| IBIS file generated by GenIBIS.pl Version 3.20?
|   centaurus
[IBIS ver]   4.1
[File name]   sprm555a.ibs
[File Rev]   1.0
[Date]   Mon Mar 12, 2012, 13:6:18
[Source]   Data created at Texas Instruments
[Notes]   Checked with IBISCHK5.0.0 with the following exceptions...
   68 warnings. These warnings can be waived.
   Models generated for the following conditions...
   Industrial temperature range -40C to 125C
   Max supply tolerance 10%
   Some pins may contain selectors which are not valid options
   for that particular pin
   Please refer to the device datasheet for information on picking
   the correct selector model, which depends on various software
   register configurations.
   Some pins are modeled as IO or tri-state for output mode
[Disclaimer] Please be aware that in the absence of a written agreement,
   Texas Instruments (TI) assumes no liability for: 1) the
   accuracy of the IBIS models provided to your company, 2) the
   proper functioning of these IBIS models in your design or for
   any resulting applications, or, 3) infringement of patents,
   copyrights, or intellectual property rights resulting from
   your use of these IBIS models. TI provides IBIS models as a
   service to our customers and therefore reserves the right to
   limit distribution of the IBIS models.
[Copyright]   Property of Texas Instruments Incorporated. Unauthorised
   reproduction and/or distribution is strictly prohibited. This
   product is protected under copyright law and trade secret law
   as an unpublished work. Created 2010,(C) Copyright 2010,
   Texas Instruments Incorporated., All Rights Reserved. These
   commodities are under the U.S. Government distribution license
   control.As such,they are not to be re-exported without the
   prior approval of the U.S. Department of Commerce.
|   Component centaurus
[Component]   centaurus
[Manufacturer]   Texas Instruments.
| Source IO level model revisions
|Model   Revision   Date
|BC1833DV40DCPBFBP18LL_SSDHH   1.1   May 27, 2010
|IQ1833DVTCKPBFBP18LL_SSDHH   1.1   May 27, 2010
|BCSHTLTCSCDVPBFZ_SSGFV   1.0   May 31, 2010
|BC1833DV40DCMLBPBFBP18LL_SSDHH   1.1   May 27, 2010
|BCSHTLTCSCDDVPBFZ_SSGFV   1.0   May 31, 2010
|BC1833DV40DCPBFBP18LL_SSDHV   1.1   May 27, 2010
|IHHV1833DVHYP18LL_SSDHH   1.1   May 27, 2010
[Package]
|   typ   min   max
R_pkg   1.068   2.06E-1   1.93E0
L_pkg   3.135E-009   9.00E-10   5.37E-9
C_pkg   2.2305E-012   6.21E-13   3.84E-12
[Pin]   signal_name   model_name   R_pin   L_pin   C_pin
R5   AUD_CLKIN1   Selector_4   9.45E-1   3.06E-9   1.21E-12
H1   AUD_CLKIN2   Selector_4   1.37E0   3.69E-9   1.87E-12
L5   AUD_CLKIN0   Selector_4   6.71E-1   2.16E-9   1.01E-12
R1   AUXOSC_MXI   NC
T1   AUXOSC_MXO   NC
AC22   CAM_D[5]   Selector_4   6.39E-1   1.94E-9   1.07E-12
AB17   CAM_D[7]   Selector_4   1.03E0   3.13E-9   1.41E-12
J7   CLKIN32   Selector_4   3.20E-1   1.40E-9   8.51E-13
AG6   DCAN0_RX   Selector_11  1.16E0   3.22E-9   1.76E-12
AH6   DCAN0_TX   Selector_11  1.31E0   3.47E-9   1.75E-12
B27   DDR[0]_VTP   NC
D2   DDR[1]_DQS[0]N   Selector_5   1.36E0   3.45E-9   1.85E-12
G18   DDR[0]_ODT[0]   Selector_9   1.23E0   3.23E-9   1.73E-12
B19   DDR[0]_A[0]   Selector_9   1.26E0   3.41E-9   1.56E-12
G12   DDR[1]_CS[0]N   Selector_9   1.13E0   3.21E-9   1.57E-12
B10   DDR[1]_A[12]   Selector_9   1.12E0   3.01E-9   1.70E-12
A22   DDR[0]_D[27]   Selector_2   1.26E0   3.33E-9   1.71E-12
B21   DDR[0]_DQS[3]   Selector_5   1.33E0   3.47E-9   1.55E-12
F14   DDR[1]_BA[0]   Selector_9   1.17E0   3.16E-9   1.49E-12
B7   DDR[1]_D[23]   Selector_2   1.30E0   3.46E-9   1.64E-12
A23   DDR[0]_DQS[2]N   Selector_5   1.43E0   3.76E-9   1.79E-12
D21   DDR[0]_D[30]   Selector_2   1.20E0   3.62E-9   1.70E-12
E26   DDR[0]_D[2]   Selector_2   1.53E0   3.78E-9   1.83E-12
F15   DDR[0]_BA[0]   Selector_9   1.25E0   3.63E-9   1.66E-12
F21   DDR[0]_D[25]   Selector_2   1.28E0   3.44E-9   1.85E-12
B17   DDR[0]_A[5]   Selector_9   1.20E0   3.20E-9   1.80E-12
C18   DDR[0]_CASN   Selector_9   1.22E0   3.31E-9   1.69E-12
A11   DDR[1]_A[11]   Selector_9   1.13E0   3.02E-9   1.56E-12
C27   DDR[0]_D[8]   Selector_2   1.55E0   4.01E-9   2.08E-12
C26   DDR[0]_D[10]   Selector_2   1.60E0   4.13E-9   2.02E-12
E28   DDR[0]_DQM[0]   Selector_9   1.55E0   3.87E-9   1.90E-12
D23   DDR[0]_D[20]   Selector_2   1.33E0   3.53E-9   1.94E-12
A3   DDR[1]_DQS[1]N   Selector_5   1.52E0   3.80E-9   1.90E-12
E2   DDR[1]_D[2]   Selector_2   1.34E0   3.62E-9   1.77E-12
C28   DDR[0]_D[7]   Selector_2   1.57E0   3.88E-9   2.07E-12
A8   DDR[1]_DQS[3]N   Selector_5   1.28E0   3.23E-9   1.64E-12
C25   DDR[0]_D[9]   Selector_2   1.57E0   3.94E-9   3.84E-12
F12   DDR[1]_A[10]   Selector_9   1.14E0   3.17E-9   1.62E-12
F5   DDR[1]_D[4]   Selector_2   1.26E0   3.20E-9   1.84E-12
C20   DDR[0]_D[28]   Selector_2   1.26E0   3.32E-9   1.78E-12
A4   DDR[1]_D[14]   Selector_2   1.43E0   3.72E-9   1.94E-12
C6   DDR[1]_D[20]   Selector_2   1.28E0   3.23E-9   1.79E-12
A26   DDR[0]_DQS[1]N   Selector_5   1.63E0   4.15E-9   1.86E-12
D5   DDR[1]_D[9]   Selector_2   1.53E0   3.76E-9   1.90E-12
B2   DDR[1]_DQM[1]   Selector_9   1.53E0   3.96E-9   1.86E-12
B11   DDR[1]_A[0]   Selector_9   1.18E0   3.24E-9   1.50E-12
A5   DDR[1]_D[15]   Selector_2   1.46E0   3.76E-9   1.87E-12
C3   DDR[1]_D[10]   Selector_2   1.55E0   3.97E-9   1.96E-12
D17   DDR[0]_A[11]   Selector_9   1.19E0   3.09E-9   1.68E-12
E18   DDR[0]_A[7]   Selector_9   1.27E0   3.80E-9   1.73E-12
G10   DDR[1]_RST   Selector_9   1.07E0   3.11E-9   1.47E-12
E4   DDR[1]_D[5]   Selector_2   1.36E0   3.56E-9   1.91E-12
F26   DDR[0]_D[1]   Selector_2   1.52E0   3.82E-9   1.92E-12
C24   DDR[0]_DQM[2]   Selector_9   1.40E0   3.60E-9   1.79E-12
A15   DDR[0]_A[6]   Selector_9   1.21E0   3.23E-9   1.79E-12
C5   DDR[1]_D[18]   Selector_2   1.33E0   3.41E-9   1.89E-12
D3   DDR[1]_D[6]   Selector_2   1.32E0   3.47E-9   1.71E-12
B6   DDR[1]_DQS[2]N   Selector_5   1.36E0   3.37E-9   1.68E-12
B13   DDR[1]_CLK   Selector_9   1.20E0   3.79E-9   1.56E-12
E17   DDR[0]_A[12]   Selector_9   1.21E0   3.55E-9   1.65E-12
B16   DDR[0]_CLK   Selector_9   1.27E0   3.88E-9   1.54E-12
G20   DDR[0]_D[26]   Selector_2   1.30E0   3.60E-9   1.82E-12
B3   DDR[1]_DQS[1]   Selector_5   1.51E0   3.78E-9   1.67E-12
F4   DDR[1]_DQM[0]   Selector_9   1.26E0   3.24E-9   1.85E-12
D1   DDR[1]_DQS[0]   Selector_5   1.38E0   3.46E-9   1.70E-12
E12   DDR[1]_WEN   Selector_9   1.17E0   3.19E-9   1.55E-12
G11   DDR[1]_CS[1]N   Selector_9   1.19E0   3.21E-9   1.63E-12
C9   DDR[1]_D[28]   Selector_2   1.18E0   2.93E-9   1.74E-12
E23   DDR[0]_D[21]   Selector_2   1.38E0   3.89E-9   1.95E-12
F9   DDR[1]_D[24]   Selector_2   1.18E0   3.06E-9   1.51E-12
E6   DDR[1]_D[21]   Selector_2   1.31E0   3.50E-9   1.96E-12
B20   DDR[0]_D[31]   Selector_2   1.28E0   3.43E-9   1.66E-12
C15   DDR[0]_A[9]   Selector_9   1.21E0   3.27E-9   1.50E-12
G8   DDR[1]_DQM[2]   Selector_9   1.31E0   3.42E-9   1.56E-12
B4   DDR[1]_D[12]   Selector_2   1.42E0   3.61E-9   2.05E-12
C21   DDR[0]_D[29]   Selector_2   1.31E0   3.59E-9   1.80E-12
A24   DDR[0]_D[15]   Selector_2   1.58E0   4.12E-9   1.99E-12
B25   DDR[0]_D[12]   Selector_2   1.52E0   3.83E-9   2.11E-12
D18   DDR[0]_A[2]   Selector_9   1.26E0   3.33E-9   1.74E-12
A9   DDR[1]_A[7]   Selector_9   1.20E0   3.36E-9   1.83E-12
B26   DDR[0]_DQS[1]   Selector_5   1.61E0   4.15E-9   1.82E-12
F3   DDR[1]_D[1]   Selector_2   1.27E0   3.39E-9   1.64E-12
H8   DDR[1]_D[16]   Selector_2   1.27E0   3.24E-9   1.61E-12
B8   DDR[1]_DQS[3]   Selector_5   1.26E0   3.17E-9   1.50E-12
H21   DDR[0]_D[18]   Selector_2   1.36E0   3.61E-9   1.75E-12
B22   DDR[0]_D[23]   Selector_2   1.36E0   3.76E-9   1.86E-12
C17   DDR[0]_WEN   Selector_9   1.25E0   3.38E-9   1.72E-12
E15   DDR[0]_A[3]   Selector_9   1.20E0   3.31E-9   1.53E-12
F16   DDR[0]_A[14]   Selector_9   1.18E0   3.06E-9   1.44E-12
G17   DDR[0]_CS[1]N   Selector_9   1.24E0   3.18E-9   1.66E-12
F25   DDR[0]_D[3]   Selector_2   1.52E0   3.77E-9   1.99E-12
A16   DDR[0]_CLKN   Selector_9   1.24E0   3.58E-9   1.59E-12
H20   DDR[0]_D[24]   Selector_2   1.26E0   3.60E-9   1.64E-12
C8   DDR[1]_D[30]   Selector_2   1.14E0   3.37E-9   1.61E-12
A6   DDR[1]_DQS[2]   Selector_5   1.38E0   3.50E-9   1.70E-12
H10   DDR[1]_ODT[0]   Selector_9   1.07E0   3.17E-9   1.41E-12
G21   DDR[0]_D[19]   Selector_2   1.33E0   3.36E-9   1.67E-12
H19   DDR[0]_ODT[1]   Selector_9   1.13E0   3.36E-9   1.53E-12
B18   DDR[0]_RASN   Selector_9   1.26E0   3.78E-9   1.79E-12
A13   DDR[1]_CLKN   Selector_9   1.17E0   3.42E-9   1.52E-12
F24   DDR[0]_D[4]   Selector_2   1.51E0   3.26E-9   1.93E-12
A25   DDR[0]_D[14]   Selector_2   1.54E0   4.00E-9   2.15E-12
E27   DDR[0]_D[0]   Selector_2   1.52E0   3.88E-9   1.81E-12
A19   DDR[0]_A[10]   Selector_9   1.21E0   3.63E-9   1.98E-12
C23   DDR[0]_D[22]   Selector_2   1.33E0   3.64E-9   1.74E-12
A21   DDR[0]_DQS[3]N   Selector_5   1.36E0   3.50E-9   1.62E-12
A10   DDR[1]_BA[1]   Selector_9   1.18E0   3.24E-9   1.75E-12
F19   DDR[0]_A[1]   Selector_9   1.21E0   3.14E-9   1.73E-12
D15   DDR[0]_A[4]   Selector_9   1.22E0   3.37E-9   1.59E-12
A14   DDR[1]_A[3]   Selector_9   1.14E0   3.29E-9   1.60E-12
C11   DDR[1]_A[2]   Selector_9   1.18E0   3.11E-9   1.71E-12
F20   DDR[0]_DQM[3]   Selector_9   1.28E0   3.28E-9   1.78E-12
A20   DDR[0]_BA[1]   Selector_9   1.25E0   3.57E-9   1.89E-12
F13   DDR[1]_CASN   Selector_9   1.15E0   2.93E-9   1.52E-12
C14   DDR[1]_A[9]   Selector_9   1.12E0   3.10E-9   1.58E-12
E3   DDR[1]_D[0]   Selector_2   1.27E0   3.46E-9   1.69E-12
B5   DDR[1]_D[19]   Selector_2   1.28E0   3.22E-9   2.06E-12
D27   DDR[0]_DQS[0]N   Selector_5   1.50E0   3.79E-9   1.95E-12
B1   DDR[1]_VTP   NC
B28   DDR[0]_DQM[1]   Selector_9   1.59E0   4.20E-9   1.98E-12
C2   DDR[1]_D[8]   Selector_2   1.48E0   3.80E-9   1.95E-12
F18   DDR[0]_CS[0]N   Selector_9   1.21E0   3.27E-9   1.72E-12
B24   DDR[0]_D[16]   Selector_2   1.36E0   3.60E-9   2.00E-12
F8   DDR[1]_D[26]   Selector_2   1.25E0   3.34E-9   1.72E-12
E11   DDR[1]_A[13]   Selector_9   1.16E0   3.23E-9   1.62E-12
B23   DDR[0]_DQS[2]   Selector_5   1.44E0   3.73E-9   1.83E-12
F10   DDR[1]_A[1]   Selector_9   1.15E0   3.10E-9   1.63E-12
A18   DDR[0]_BA[2]   Selector_9   1.19E0   3.57E-9   1.75E-12
A27   DDR[0]_D[11]   Selector_2   1.55E0   3.94E-9   2.00E-12
A7   DDR[1]_D[27]   Selector_2   1.20E0   2.99E-9   1.70E-12
B9   DDR[1]_D[31]   Selector_2   1.21E0   3.14E-9   1.64E-12
D11   DDR[1]_A[14]   Selector_9   1.13E0   3.04E-9   1.53E-12
G9   DDR[1]_DQM[3]   Selector_9   1.20E0   3.12E-9   1.48E-12
D6   DDR[1]_D[22]   Selector_2   1.27E0   3.43E-9   1.86E-12
F17   DDR[0]_A[13]   Selector_9   1.23E0   3.22E-9   1.74E-12
C1   DDR[1]_D[7]   Selector_2   1.33E0   3.40E-9   1.87E-12
D14   DDR[1]_A[6]   Selector_9   1.18E0   3.14E-9   1.50E-12
F11   DDR[1]_ODT[1]   Selector_9   1.18E0   3.30E-9   1.54E-12
D28   DDR[0]_DQS[0]   Selector_5   1.51E0   3.84E-9   1.68E-12
C12   DDR[1]_RASN   Selector_9   1.20E0   3.36E-9   1.65E-12
F7   DDR[1]_D[17]   Selector_2   1.33E0   3.38E-9   1.77E-12
H9   DDR[1]_D[25]   Selector_2   1.22E0   3.29E-9   1.77E-12
F22   DDR[0]_D[17]   Selector_2   1.39E0   3.53E-9   1.87E-12
B12   DDR[1]_A[5]   Selector_9   1.13E0   3.03E-9   1.59E-12
H11   DDR[1]_CKE   Selector_9   1.09E0   3.30E-9   1.54E-12
A2   DDR[1]_D[11]   Selector_2   1.51E0   3.71E-9   2.02E-12
C4   DDR[1]_D[13]   Selector_2   1.49E0   3.88E-9   2.05E-12
B14   DDR[1]_A[4]   Selector_9   1.14E0   3.37E-9   1.65E-12
E1   DDR[1]_D[3]   Selector_2   1.30E0   3.25E-9   1.69E-12
E14   DDR[1]_A[8]   Selector_9   1.17E0   3.23E-9   1.61E-12
G19   DDR[0]_RST   Selector_9   1.13E0   3.36E-9   1.61E-12
H18   DDR[0]_CKE   Selector_9   1.15E0   3.45E-9   1.63E-12
B15   DDR[0]_A[8]   Selector_9   1.26E0   3.50E-9   1.49E-12
D24   DDR[0]_D[13]   Selector_2   1.58E0   4.13E-9   2.13E-12
D12   DDR[1]_BA[2]   Selector_9   1.14E0   3.10E-9   1.76E-12
D26   DDR[0]_D[6]   Selector_2   1.53E0   3.79E-9   1.87E-12
E25   DDR[0]_D[5]   Selector_2   1.56E0   3.85E-9   1.90E-12
D8   DDR[1]_D[29]   Selector_2   1.24E0   3.51E-9   1.57E-12
AH2   DEVOSC_MXI   NC
AH3   DEVOSC_MXO   NC
W6   DEVOSC_WAKE   Selector_4   1.18E0   3.40E-9   1.79E-12
R23   EMAC[0]_MRXD[2]   Selector_4   1.24E0   3.55E-9   1.90E-12
L23   EMAC[0]_MCOL   Selector_4   5.15E-1   1.64E-9   9.49E-13
H22   EMAC[0]_MTXD[2]   Selector_4   1.00E0   2.82E-9   1.33E-12
J22   EMAC[0]_MTXD[6]   Selector_4   8.58E-1   2.59E-9   1.29E-12
J26   EMAC[0]_MRXER   Selector_4   8.69E-1   2.53E-9   1.22E-12
K22   EMAC[0]_MRXDV   Selector_4   7.90E-1   2.39E-9   1.28E-12
J27   EMAC_RMREFCLK   Selector_4   1.08E0   3.17E-9   1.40E-12
H23   EMAC[0]_MTXD[3]   Selector_4   1.02E0   2.91E-9   1.48E-12
T23   EMAC[0]_MRXD[4]   Selector_4   1.33E0   3.72E-9   1.76E-12
F28   EMAC[0]_MRXD[6]   Selector_4   1.30E0   3.58E-9   1.72E-12
J25   EMAC[0]_MRXD[3]   Selector_4   7.51E-1   2.18E-9   1.24E-12
R25   EMAC[0]_MCRS   Selector_4   1.36E0   3.81E-9   1.66E-12
J23   EMAC[0]_MTXEN   Selector_4   5.73E-1   1.75E-9   1.09E-12
F27   EMAC[0]_MTXD[5]   Selector_4   1.14E0   3.17E-9   1.79E-12
H27   EMAC[0]_MRCLK   Selector_4   1.07E0   3.03E-9   1.35E-12
L24   EMAC[0]_MTCLK   Selector_4   6.57E-1   1.98E-9   1.11E-12
G27   EMAC[0]_MRXD[7]   Selector_4   1.10E0   3.05E-9   1.47E-12
H25   EMAC[0]_MTXD[1]   Selector_4   9.03E-1   2.62E-9   1.31E-12
K23   EMAC[0]_GMTCLK   Selector_4   4.74E-1   1.67E-9   9.00E-13
J24   EMAC[0]_MTXD[0]   Selector_4   6.71E-1   2.13E-9   1.04E-12
P23   EMAC[0]_MRXD[1]   Selector_4   9.64E-1   3.09E-9   1.29E-12
G23   EMAC[0]_MTXD[4]   Selector_4   1.05E0   2.99E-9   1.64E-12
H24   EMAC[0]_MTXD[7]   Selector_4   7.06E-1   2.19E-9   1.19E-12
H26   EMAC[0]_MRXD[5]   Selector_4   9.44E-1   2.78E-9   1.47E-12
G28   EMAC[0]_MRXD[0]   Selector_4   1.26E0   3.34E-9   1.63E-12
AG8   EMU0   Selector_11  1.70E0   4.77E-9   1.95E-12
AE11   EMU1   Selector_11  1.27E0   3.77E-9   1.75E-12
AB28   GPMC_D[9]   Selector_4   1.44E0   3.90E-9   1.94E-12
AE28   GPMC_A[18]   Selector_4   1.51E0   4.38E-9   1.95E-12
V23   GPMC_A[17]   Selector_4   6.27E-1   2.03E-9   1.20E-12
AD27   GPMC_A[16]   Selector_4   1.46E0   3.72E-9   1.96E-12
U23   GPMC_D[13]   Selector_4   5.80E-1   1.78E-9   1.06E-12
M26   GPMC_ADVN_ALE   Selector_4   1.19E0   3.50E-9   1.84E-12
AD28   GPMC_A[20]   Selector_4   1.54E0   4.14E-9   2.05E-12
AC28   GPMC_A[21]   Selector_4   1.44E0   4.27E-9   1.92E-12
U26   GPMC_D[0]   Selector_4   8.82E-1   2.85E-9   1.29E-12
Y27   GPMC_D[8]   Selector_4   1.23E0   3.53E-9   1.73E-12
T27   GPMC_OEN_REN   Selector_4   1.00E0   2.82E-9   1.57E-12
AC27   GPMC_A[19]   Selector_4   1.36E0   3.90E-9   1.75E-12
V26   GPMC_D[4]   Selector_4   1.06E0   3.00E-9   1.56E-12
V24   GPMC_D[14]   Selector_4   7.73E-1   2.39E-9   1.21E-12
Y26   GPMC_D[10]   Selector_4   1.02E0   2.85E-9   1.52E-12
U25   GPMC_D[6]   Selector_4   8.49E-1   2.48E-9   1.35E-12
W28   GPMC_WAIT[0]   Selector_4   1.32E0   3.52E-9   1.72E-12
U28   GPMC_WEN   Selector_4   1.22E0   3.45E-9   1.64E-12
AB27   GPMC_A[22]   Selector_4   1.28E0   3.70E-9   1.88E-12
R26   GPMC_CLK   Selector_4   8.74E-1   2.46E-9   1.37E-12
M25   GPMC_CS[2]N   Selector_4   7.19E-1   2.25E-9   1.46E-12
AA28   GPMC_D[5]   Selector_4   1.41E0   3.90E-9   1.97E-12
P25   GPMC_CS[4]N   Selector_4   1.26E0   3.40E-9   1.56E-12
V27   GPMC_D[2]   Selector_4   1.15E0   3.34E-9   1.59E-12
U27   GPMC_BE[0]N_CLE   Selector_4   1.07E0   3.10E-9   1.61E-12
T28   GPMC_CS[0]N   Selector_4   1.82E0   4.91E-9   2.18E-12
U24   GPMC_D[12]   Selector_4   7.10E-1   2.16E-9   1.22E-12
K28   GPMC_CS[1]N   Selector_4   1.34E0   3.33E-9   1.67E-12
V25   GPMC_D[7]   Selector_4   8.64E-1   2.75E-9   1.13E-12
AA26   GPMC_A[23]   Selector_4   1.03E0   3.09E-9   1.59E-12
W27   GPMC_D[3]   Selector_4   1.25E0   3.42E-9   1.67E-12
V28   GPMC_BE[1]N   Selector_4   1.27E0   3.39E-9   1.63E-12
Y25   GPMC_D[15]   Selector_4   9.86E-1   2.75E-9   1.42E-12
Y28   GPMC_D[1]   Selector_4   1.36E0   3.79E-9   1.76E-12
P26   GPMC_CS[3]N   Selector_4   1.32E0   3.69E-9   1.74E-12
AA27   GPMC_D[11]   Selector_4   1.23E0   3.40E-9   1.68E-12
G6   MCA[3]_ACLKX   Selector_4   1.19E0   3.43E-9   1.64E-12
M4   MCA[0]_AXR[6]   Selector_4   6.90E-1   2.20E-9   1.11E-12
N6   MCA[1]_AXR[3]   Selector_4   3.91E-1   1.58E-9   8.55E-13
M6   MCA[0]_AXR[9]   Selector_4   4.26E-1   1.74E-9   1.01E-12
J4   MCA[4]_AXR[1]   Selector_4   9.89E-1   2.89E-9   1.32E-12
H5   MCA[5]_AFSX   Selector_4   1.27E0   3.56E-9   1.84E-12
L1   MCA[0]_AXR[8]   Selector_4   1.09E0   3.11E-9   1.51E-12
H4   MCA[3]_AFSX   Selector_4   8.85E-1   2.60E-9   1.35E-12
L4   MCA[0]_AXR[2]   Selector_4   7.39E-1   2.46E-9   1.21E-12
L3   MCA[0]_AFSX   Selector_4   8.34E-1   2.46E-9   1.33E-12
K1   MCA[0]_AFSR   Selector_4   1.09E0   3.04E-9   1.52E-12
V3   MCA[1]_AFSX   Selector_4   1.69E0   4.83E-9   2.01E-12
J3   MCA[5]_ACLKX   Selector_4   8.04E-1   2.45E-9   1.47E-12
R4   MCA[0]_ACLKX   Selector_4   1.06E0   3.15E-9   1.50E-12
J6   MCA[3]_AXR[3]   Selector_4   6.01E-1   1.98E-9   1.16E-12
U6   MCA[2]_ACLKX   Selector_4   9.32E-1   2.90E-9   1.28E-12
N2   MCA[2]_AXR[0]   Selector_4   8.59E-1   2.52E-9   1.37E-12
H6   MCA[4]_AXR[0]   Selector_4   1.17E0   3.17E-9   1.61E-12
R6   MCA[0]_AXR[4]   Selector_4   8.02E-1   2.45E-9   1.27E-12
K7   MCA[4]_ACLKX   Selector_4   3.11E-1   1.44E-9   8.81E-13
M5   MCA[0]_AXR[3]   Selector_4   5.38E-1   1.93E-9   1.04E-12
H2   MCA[2]_AXR[3]   Selector_4   1.25E0   3.57E-9   1.71E-12
L7   MCA[5]_AXR[0]   Selector_4   3.14E-1   1.39E-9   7.88E-13
J2   MCA[0]_AXR[0]   Selector_4   1.06E0   3.00E-9   1.53E-12
AA5   MCA[2]_AFSX   Selector_4   1.77E0   5.15E-9   2.14E-12
M3   MCA[0]_AXR[5]   Selector_4   6.82E-1   2.23E-9   1.29E-12
R3   MCA[1]_AXR[2]   Selector_4   1.00E0   3.03E-9   1.31E-12
V4   MCA[1]_AXR[0]   Selector_4   1.62E0   4.67E-9   1.93E-12
U5   MCA[1]_ACLKX   Selector_4   1.21E0   3.49E-9   1.49E-12
G1   MCA[3]_AXR[0]   Selector_4   1.16E0   3.34E-9   1.66E-12
J1   MCA[0]_AXR[1]   Selector_4   1.31E0   3.77E-9   1.60E-12
V6   MCA[2]_AXR[1]   Selector_4   1.21E0   3.48E-9   1.52E-12
L6   MCA[5]_AXR[1]   Selector_4   5.44E-1   1.94E-9   1.02E-12
H3   MCA[4]_AFSX   Selector_4   9.61E-1   2.78E-9   1.49E-12
F2   MCA[3]_AXR[2]   Selector_4   1.24E0   3.47E-9   1.81E-12
K2   MCA[0]_ACLKR   Selector_4   1.07E0   3.00E-9   1.51E-12
T6   MCA[1]_AXR[1]   Selector_4   6.28E-1   2.09E-9   1.16E-12
G2   MCA[3]_AXR[1]   Selector_4   1.09E0   3.15E-9   1.62E-12
M1   MCA[1]_ACLKR   Selector_4   1.06E0   3.13E-9   1.40E-12
M2   MCA[1]_AFSR   Selector_4   1.01E0   2.88E-9   1.44E-12
L2   MCA[0]_AXR[7]   Selector_4   1.04E0   2.82E-9   1.44E-12
V5   MCA[2]_AXR[2]   Selector_4   1.30E0   3.96E-9   1.72E-12
H28   MDCLK   Selector_4   1.16E0   3.25E-9   1.72E-12
P24   MDIO   Selector_4   1.06E0   3.29E-9   1.42E-12
H7   NMIN   Selector_1   9.93E-1   2.99E-9   1.47E-12
F1   PORN   Selector_12  1.37E0   3.48E-9   1.78E-12
J5   RESETN   Selector_1   7.19E-1   2.26E-9   1.13E-12
K6   RSTOUTN_WDN_OUTN   Selector_3   5.10E-1   1.65E-9   9.95E-13
AD4   RTCK   Selector_10  1.01E0   2.73E-9   1.35E-12
Y4   SD0_DAT[3]   Selector_4   1.65E0   4.91E-9   2.04E-12
Y6   SD0_CLK   Selector_4   1.41E0   4.09E-9   1.76E-12
N1   SD0_CMD   Selector_4   1.11E0   3.25E-9   1.48E-12
Y3   SD0_DAT[2]_SDRWN   Selector_4   1.77E0   5.01E-9   2.33E-12
R7   SD0_DAT[0]   Selector_4   3.52E-1   1.36E-9   8.89E-13
Y5   SD0_DAT[1]_SDIRQN   Selector_4   1.54E0   4.43E-9   2.06E-12
P3   SD1_CLK   Selector_3   8.83E-1   2.54E-9   1.28E-12
P6   SD1_DAT[3]   Selector_4   5.29E-1   1.77E-9   9.16E-13
P1   SD1_DAT[0]   Selector_4   1.05E0   2.94E-9   1.43E-12
P5   SD1_DAT[1]_SDIRQN   Selector_4   6.41E-1   2.18E-9   9.48E-13
P4   SD1_DAT[2]_SDRWN   Selector_4   7.18E-1   2.35E-9   1.12E-12
P2   SD1_CMD   Selector_4   9.71E-1   2.85E-9   1.75E-12
L25   SD2_DAT[7]   Selector_4   7.41E-1   2.31E-9   1.18E-12
K27   SD2_DAT[2]_SDRWN   Selector_4   1.08E0   3.10E-9   1.51E-12
M23   SD2_SCLK   Selector_4   5.06E-1   1.67E-9   8.92E-13
M24   SD2_DAT[1]_SDIRQN   Selector_4   5.74E-1   1.89E-9   9.89E-13
L26   SD2_DAT[0]   Selector_4   9.09E-1   2.58E-9   1.29E-12
R24   SD2_DAT[4]   Selector_4   1.07E0   3.12E-9   1.52E-12
N23   SD2_DAT[6]   Selector_4   5.87E-1   2.07E-9   1.02E-12
J28   SD2_DAT[3]   Selector_4   1.17E0   3.18E-9   1.57E-12
P22   SD2_DAT[5]   Selector_4   6.18E-1   2.06E-9   1.05E-12
AD6   SPI[0]_SCS[0]N   Selector_11  8.21E-1   2.38E-9   1.33E-12
AF3   SPI[0]_D[1]   Selector_11  1.25E0   3.81E-9   1.77E-12
AD3   SPI[1]_SCS[0]N   Selector_11  1.18E0   3.37E-9   1.69E-12
AA3   SPI[1]_D[1]   Selector_11  1.26E0   3.76E-9   1.76E-12
AC3   SPI[1]_SCLK   Selector_11  1.15E0   3.22E-9   1.60E-12
AC7   SPI[0]_SCLK   Selector_11  7.08E-1   2.19E-9   1.09E-12
AE5   SPI[0]_SCS[1]N   Selector_11  1.02E0   3.18E-9   1.41E-12
AA6   SPI[1]_D[0]   Selector_11  9.30E-1   2.78E-9   1.49E-12
AE3   SPI[0]_D[0]   Selector_11  1.26E0   3.49E-9   1.76E-12
W7   TCLK   Selector_8   5.20E-1   1.72E-9   9.01E-13
T2   TCLKIN   Selector_7   9.60E-1   2.66E-9   1.33E-12
Y7   TDI   Selector_6   8.98E-1   2.78E-9   1.44E-12
AC5   TDO   Selector_3   7.43E-1   2.13E-9   1.08E-12
AA7   TMS   Selector_1   5.16E-1   1.56E-9   9.14E-13
AA4   TRSTN   Selector_1   9.21E-1   2.56E-9   1.27E-12
AF5   UART0_RTSN   Selector_11  1.13E0   3.73E-9   1.53E-12
AH4   UART0_DCDN   Selector_11  1.35E0   3.74E-9   1.80E-12
AE6   UART0_CTSN   Selector_11  1.00E0   2.80E-9   1.47E-12
AG2   UART0_DTRN   Selector_11  1.46E0   3.89E-9   1.96E-12
AG5   UART0_TXD   Selector_10  1.22E0   3.29E-9   1.74E-12
AF4   UART0_RIN   Selector_11  1.24E0   3.23E-9   1.73E-12
AH5   UART0_RXD   Selector_6   1.38E0   3.54E-9   1.79E-12
AG4   UART0_DSRN   Selector_11  1.31E0   3.62E-9   1.80E-12
U4   UART2_RXD   Selector_7   6.85E-1   2.04E-9   1.16E-12
U3   UART2_TXD   Selector_7   9.31E-1   2.65E-9   1.32E-12
AH8   VIN[0]A_D[4]   Selector_11  1.73E0   4.86E-9   2.37E-12
AB20   VIN[0]A_CLK   Selector_11  4.67E-1   1.63E-9   8.90E-13
AH16   VIN[0]A_D[6]   Selector_11  1.13E0   3.05E-9   1.36E-12
AC20   VIN[0]A_HSYNC   Selector_11  5.37E-1   1.76E-9   9.21E-13
AF17   VIN[0]A_D[13]_BD[5]  Selector_11  7.77E-1   2.45E-9   1.33E-12
AA21   VIN[0]A_D[16]   Selector_4   2.06E-1   9.00E-10   6.21E-13
AD20   VIN[0]A_VSYNC   Selector_11  5.69E-1   1.74E-9   1.12E-12
AF9   VIN[0]A_D[0]   Selector_11  1.65E0   4.87E-9   2.00E-12
AB15   VIN[0]A_D[8]_BD[0]   Selector_11  6.48E-1   2.10E-9   1.11E-12
AC21   VIN[0]A_D[22]   Selector_4   5.25E-1   1.69E-9   9.56E-13
AC12   VIN[0]A_D[14]_BD[6]  Selector_11  1.39E0   4.00E-9   1.65E-12
AE18   VIN[0]A_D[21]   Selector_4   1.09E0   3.15E-9   1.48E-12
AE21   VIN[0]A_DE   Selector_11  8.59E-1   2.54E-9   1.28E-12
AF20   VIN[0]A_D[18]   Selector_4   9.07E-1   2.61E-9   1.42E-12
AC14   VIN[0]A_D[15]_BD[7]  Selector_11  9.28E-1   2.74E-9   1.45E-12
AA11   VIN[0]A_D[7]   Selector_11  9.56E-1   2.86E-9   1.37E-12
AG17   VIN[0]A_D[12]_BD[4]  Selector_11  9.68E-1   2.98E-9   1.52E-12
AB11   VIN[0]A_D[1]   Selector_11  1.10E0   3.24E-9   1.59E-12
AG16   VIN[0]A_D[5]   Selector_11  9.22E-1   2.76E-9   1.42E-12
AE12   VIN[0]A_D[3]   Selector_11  1.15E0   3.70E-9   1.73E-12
AB21   VIN[0]A_D[17]   Selector_4   3.27E-1   1.32E-9   7.89E-13
AE17   VIN[0]B_CLK   Selector_11  1.08E0   3.16E-9   1.61E-12
AC17   VIN[0]A_D[20]   Selector_4   9.04E-1   2.79E-9   1.35E-12
AG9   VIN[0]A_D[9]_BD[1]   Selector_11  1.73E0   4.80E-9   2.21E-12
AH17   VIN[0]A_D[11]_BD[3]  Selector_11  1.14E0   3.37E-9   1.56E-12
AA20   VIN[0]A_FLD   Selector_11  3.16E-1   1.20E-9   7.09E-13
AD17   VIN[0]B_FLD   Selector_4   1.33E0   3.66E-9   1.65E-12
AF21   VIN[0]A_D[19]   Selector_4   9.56E-1   2.77E-9   1.46E-12
AC9   VIN[0]A_D[2]   Selector_11  1.43E0   3.96E-9   1.91E-12
AC15   VIN[0]B_DE   Selector_4   1.40E0   3.92E-9   1.75E-12
AC16   VIN[0]A_D[23]   Selector_4   9.46E-1   2.74E-9   1.28E-12
AH9   VIN[0]A_D[10]_BD[2]  Selector_11  1.79E0   5.09E-9   2.32E-12
AE14   VOUT[0]_G_Y_YC[8]   Selector_10  8.04E-1   2.44E-9   1.19E-12
AH7   VOUT[0]_G_Y_YC[2]   Selector_11  1.93E0   5.37E-9   2.28E-12
AE23   VOUT[1]_B_CB_C[1]   Selector_4   1.03E0   2.93E-9   1.31E-12
AF27   VOUT[1]_G_Y_YC[2]   Selector_4   1.61E0   4.28E-9   2.23E-12
AE26   VOUT[1]_G_Y_YC[8]   Selector_4   1.37E0   3.86E-9   1.99E-12
AD14   VOUT[0]_G_Y_YC[7]   Selector_10  6.42E-1   2.10E-9   1.11E-12
Y24   VOUT[1]_R_CR[9]   Selector_4   7.60E-1   2.30E-9   1.18E-12
AC24   VOUT[1]_HSYNC   Selector_4   7.83E-1   2.40E-9   1.33E-12
AF18   VOUT[0]_FLD   Selector_4   1.38E0   3.80E-9   1.71E-12
AE15   VOUT[0]_B_CB_C[3]   Selector_11  7.36E-1   2.26E-9   1.13E-12
AB9   VOUT[0]_R_CR[3]   Selector_11  9.83E-1   3.02E-9   1.36E-12
AC11   VOUT[0]_HSYNC   Selector_10  1.08E0   3.23E-9   1.44E-12
AG26   VOUT[1]_G_Y_YC[5]   Selector_4   1.54E0   4.35E-9   2.07E-12
Y23   VOUT[1]_G_Y_YC[3]   Selector_4   5.65E-1   1.91E-9   1.11E-12
AG28   VOUT[1]_R_CR[3]   Selector_4   1.75E0   4.64E-9   2.18E-12
AB10   VOUT[0]_B_CB_C[7]   Selector_10  1.01E0   3.09E-9   1.41E-12
AE27   VOUT[1]_R_CR[2]   Selector_4   1.53E0   4.13E-9   2.03E-12
AA25   VOUT[1]_R_CR[6]   Selector_4   9.55E-1   2.72E-9   1.42E-12
AA9   VOUT[0]_R_CR[4]   Selector_10  1.02E0   2.74E-9   1.45E-12
AE8   VOUT[0]_R_CR[8]   Selector_10  1.32E0   3.73E-9   1.81E-12
AF26   VOUT[1]_G_Y_YC[7]   Selector_4   1.44E0   3.93E-9   1.83E-12
AA10   VOUT[0]_AVID   Selector_11  9.05E-1   2.70E-9   1.36E-12
AC25   VOUT[1]_B_CB_C[7]   Selector_4   1.02E0   3.18E-9   1.48E-12
AD12   VOUT[0]_CLK   Selector_10  1.08E0   3.11E-9   1.52E-12
AB23   VOUT[1]_FLD   Selector_4   7.19E-1   2.16E-9   1.04E-12
AA8   VOUT[0]_G_Y_YC[6]   Selector_10  9.40E-1   2.96E-9   1.32E-12
AG7   VOUT[0]_B_CB_C[2]   Selector_11  1.67E0   4.70E-9   2.29E-12
W23   VOUT[1]_R_CR[8]   Selector_4   6.12E-1   1.96E-9   1.16E-12
AF25   VOUT[1]_B_CB_C[5]   Selector_4   1.30E0   3.47E-9   1.80E-12
AF14   VOUT[0]_G_Y_YC[9]   Selector_10  8.54E-1   2.59E-9   1.15E-12
AF6   VOUT[0]_R_CR[6]   Selector_10  1.79E0   5.04E-9   2.20E-12
AG25   VOUT[1]_B_CB_C[4]   Selector_4   1.46E0   3.82E-9   1.96E-12
W22   VOUT[1]_G_Y_YC[4]   Selector_4   3.79E-1   1.38E-9   9.41E-13
AF15   VOUT[0]_B_CB_C[8]   Selector_10  8.55E-1   2.61E-9   1.26E-12
AC10   VOUT[0]_B_CB_C[6]   Selector_10  1.11E0   3.24E-9   1.54E-12
AD25   VOUT[1]_B_CB_C[6]   Selector_4   1.11E0   3.16E-9   1.54E-12
AA22   VOUT[1]_R_CR[0]   Selector_4   4.73E-1   1.49E-9   1.04E-12
AH15   VOUT[0]_G_Y_YC[3]   Selector_11  1.09E0   3.13E-9   1.56E-12
AC26   VOUT[1]_R_CR[5]   Selector_4   1.18E0   3.38E-9   1.62E-12
AB8   VOUT[0]_G_Y_YC[4]   Selector_10  1.26E0   3.66E-9   1.77E-12
AC13   VOUT[0]_R_CR[9]   Selector_10  5.66E-1   1.80E-9   1.09E-12
AF8   VOUT[0]_R_CR[5]   Selector_10  1.42E0   3.89E-9   1.85E-12
AB12   VOUT[0]_G_Y_YC[5]   Selector_10  6.75E-1   2.18E-9   1.08E-12
AD11   VOUT[0]_B_CB_C[4]   Selector_10  1.14E0   3.56E-9   1.54E-12
AD23   VOUT[1]_B_CB_C[0]   Selector_4   9.90E-1   2.65E-9   1.29E-12
AG27   VOUT[1]_R_CR[4]   Selector_4   1.65E0   4.42E-9   2.24E-12
AA23   VOUT[1]_VSYNC   Selector_4   6.19E-1   1.92E-9   1.09E-12
AG15   VOUT[0]_B_CB_C[9]   Selector_10  1.03E0   3.17E-9   1.43E-12
AA24   VOUT[1]_B_CB_C[9]   Selector_4   8.07E-1   2.43E-9   1.24E-12
Y22   VOUT[1]_AVID   Selector_4   5.24E-1   1.58E-9   1.02E-12
AF12   VOUT[0]_R_CR[7]   Selector_10  8.96E-1   2.70E-9   1.34E-12
AH25   VOUT[1]_B_CB_C[3]   Selector_4   1.50E0   4.11E-9   1.93E-12
AD9   VOUT[0]_R_CR[2]   Selector_11  1.25E0   3.63E-9   1.68E-12
AH26   VOUT[1]_B_CB_C[8]   Selector_4   1.60E0   4.29E-9   1.91E-12
AC19   VOUT[1]_R_CR[1]   Selector_4   1.08E0   2.98E-9   1.42E-12
AD18   VOUT[1]_G_Y_YC[1]   Selector_4   1.45E0   4.00E-9   1.84E-12
AC18   VOUT[1]_G_Y_YC[0]   Selector_4   1.37E0   3.88E-9   1.74E-12
AD15   VOUT[0]_B_CB_C[5]   Selector_10  6.31E-1   2.13E-9   1.06E-12
AD26   VOUT[1]_G_Y_YC[9]   Selector_4   1.16E0   3.37E-9   1.80E-12
AE24   VOUT[1]_CLK   Selector_4   1.08E0   3.04E-9   1.62E-12
V22   VOUT[1]_R_CR[7]   Selector_4   5.08E-1   1.57E-9   8.43E-13
AH27   VOUT[1]_G_Y_YC[6]   Selector_4   1.74E0   4.63E-9   2.36E-12
AB13   VOUT[0]_VSYNC   Selector_10  7.62E-1   2.37E-9   1.11E-12
AF28   VOUT1_B_CB_C[2]   Selector_4   1.78E0   4.36E-9   2.27E-12
[Diff Pin] inv_pin vdiff   tdelay_typ
D28   D27   200m   NA
B26   A26   200m   NA
B23   A23   200m   NA
B21   A21   200m   NA
D1   D2   200m   NA
B3   A3   200m   NA
A6   B6   200m   NA
B8   A8   200m   NA
|   Usage INPUT#1.8/3.3#X#X#BC1833DV40DCPBFBP18LL_SSDHH.PAD
|   Base model BC1833DV40DCPBFBP18LL_SSDHH
[Model Selector] Selector_1
Model_13 I/O,1.8V,Pull-up/down off,slow,IND,10%
Model_14 I/O,1.8V,Pull-down,fast,IND,10%
Model_15 I/O,1.8V,Pull-down,slow,IND,10%
Model_16 I/O,1.8V,Pull-up,fast,IND,10%
Model_17 I/O,1.8V,Pull-up/down off,fast,IND,10%
Model_18 I/O,1.8V,Pull-up,slow,IND,10%
Model_19 I/O,3.3V,Pull-up/down off,slow,IND,10%
Model_20 I/O,3.3V,Pull-down,fast,IND,10%
Model_21 I/O,3.3V,Pull-down,slow,IND,10%
Model_22 I/O,3.3V,Pull-up,fast,IND,10%
Model_23 I/O,3.3V,Pull-up/down off,fast,IND,10%
Model_24 I/O,3.3V,Pull-up,slow,IND,10%
|   Usage I/O#1.5/1.8#X#X#BCSHTLTCSCDVPBFZ_SSGFV.PAD
|   Base model BCSHTLTCSCDVPBFZ_SSGFV
[Model Selector] Selector_2
Model_100 3-STATE,1.5V,SLOWEST, 7MA,IND,10%
Model_101 3-STATE,1.5V,slow, 10MA,IND,10%
Model_102 3-STATE,1.5V,SLOWEST, 6MA,IND,10%
Model_103 3-STATE,1.5V,slow, 8MA,IND,10%
Model_104 3-STATE,1.5V,slow, 5MA,IND,10%
Model_105 3-STATE,1.5V,SLOWEST, 11MA,IND,10%
Model_106 3-STATE,1.5V,SLOWEST, 10MA,IND,10%
Model_107 3-STATE,1.5V,slow, 9MA,IND,10%
Model_108 3-STATE,1.5V,slow, 12MA,IND,10%
Model_125 3-STATE,1.8V,fast, 12MA,IND,10%
Model_126 3-STATE,1.8V,FASTEST, 5MA,IND,10%
Model_127 3-STATE,1.8V,FASTEST, 9MA,IND,10%
Model_128 3-STATE,1.8V,fast, 5MA,IND,10%
Model_129 3-STATE,1.8V,FASTEST, 7MA,IND,10%
Model_130 3-STATE,1.8V,FASTEST, 6MA,IND,10%
Model_131 3-STATE,1.8V,fast, 9MA,IND,10%
Model_132 3-STATE,1.8V,FASTEST, 11MA,IND,10%
Model_133 3-STATE,1.8V,fast, 7MA,IND,10%
Model_134 3-STATE,1.8V,FASTEST, 10MA,IND,10%
Model_135 3-STATE,1.8V,fast, 6MA,IND,10%
Model_136 3-STATE,1.8V,FASTEST, 8MA,IND,10%
Model_137 3-STATE,1.8V,fast, 11MA,IND,10%
Model_138 3-STATE,1.8V,fast, 10MA,IND,10%
Model_139 3-STATE,1.8V,FASTEST, 12MA,IND,10%
Model_140 3-STATE,1.8V,fast, 8MA,IND,10%
Model_157 3-STATE,1.5V,fast, 12MA,IND,10%
Model_158 3-STATE,1.5V,FASTEST, 5MA,IND,10%
Model_159 3-STATE,1.5V,FASTEST, 9MA,IND,10%
Model_160 3-STATE,1.5V,fast, 5MA,IND,10%
Model_161 3-STATE,1.5V,FASTEST, 7MA,IND,10%
Model_162 3-STATE,1.5V,FASTEST, 6MA,IND,10%
Model_163 3-STATE,1.5V,fast, 9MA,IND,10%
Model_164 3-STATE,1.5V,FASTEST, 11MA,IND,10%
Model_165 3-STATE,1.5V,fast, 7MA,IND,10%
Model_166 3-STATE,1.5V,FASTEST, 10MA,IND,10%
Model_167 3-STATE,1.5V,fast, 6MA,IND,10%
Model_168 3-STATE,1.5V,FASTEST, 8MA,IND,10%
Model_169 3-STATE,1.5V,fast, 11MA,IND,10%
Model_170 3-STATE,1.5V,fast, 10MA,IND,10%
Model_171 3-STATE,1.5V,FASTEST, 12MA,IND,10%
Model_172 3-STATE,1.5V,fast, 9MA,IND,10%
Model_189 INPUT,1.8V,HALFTERM, 12MA,IND,10%
Model_190 INPUT,1.8V,Pull-up/down off,IND,10%
Model_191 INPUT,1.8V,Pull-down,IND,10%
Model_192 INPUT,1.8V,FULLTERM, 5MA,IND,10%
Model_193 INPUT,1.8V,HALFTERM, 5MA,IND,10%
Model_194 INPUT,1.8V,Pull-up,IND,10%
Model_195 INPUT,1.8V,FULLTERM, 9MA,IND,10%
Model_196 INPUT,1.8V,FULLTERM, 7MA,IND,10%
Model_197 INPUT,1.8V,HALFTERM, 9MA,IND,10%
Model_198 INPUT,1.8V,FULLTERM, 6MA,IND,10%
Model_199 INPUT,1.8V,HALFTERM, 7MA,IND,10%
Model_200 INPUT,1.8V,HALFTERM, 6MA,IND,10%
Model_201 INPUT,1.8V,FULLTERM, 11MA,IND,10%
Model_202 INPUT,1.8V,Pull-up/down off,IND,10%
Model_203 INPUT,1.8V,FULLTERM, 10MA,IND,10%
Model_204 INPUT,1.8V,HALFTERM, 11MA,IND,10%
Model_205 INPUT,1.8V,FULLTERM, 8MA,IND,10%
Model_206 INPUT,1.8V,HALFTERM, 10MA,IND,10%
Model_207 INPUT,1.8V,Pull-down,IND,10%
Model_208 INPUT,1.8V,HALFTERM, 8MA,IND,10%
Model_209 INPUT,1.8V,Pull-up,IND,10%
Model_210 INPUT,1.8V,FULLTERM, 12MA,IND,10%
Model_233 INPUT,1.5V,FULLTERM, 7MA,IND,10%
Model_234 INPUT,1.5V,FULLTERM, 6MA,IND,10%
Model_235 INPUT,1.5V,HALFTERM, 12MA,IND,10%
Model_236 INPUT,1.5V,FULLTERM, 5MA,IND,10%
Model_237 INPUT,1.5V,Pull-up,IND,10%
Model_238 INPUT,1.5V,HALFTERM, 11MA,IND,10%
Model_239 INPUT,1.5V,HALFTERM, 10MA,IND,10%
Model_240 INPUT,1.5V,HALFTERM, 8MA,IND,10%
Model_241 INPUT,1.5V,FULLTERM, 12MA,IND,10%
Model_242 INPUT,1.5V,HALFTERM, 9MA,IND,10%
Model_243 INPUT,1.5V,Pull-up/down off,IND,10%
Model_244 INPUT,1.5V,HALFTERM, 7MA,IND,10%
Model_245 INPUT,1.5V,HALFTERM, 6MA,IND,10%
Model_246 INPUT,1.5V,FULLTERM, 11MA,IND,10%
Model_247 INPUT,1.5V,FULLTERM, 10MA,IND,10%
Model_248 INPUT,1.5V,Pull-down,IND,10%
Model_249 INPUT,1.5V,FULLTERM, 8MA,IND,10%
Model_250 INPUT,1.5V,HALFTERM, 5MA,IND,10%
Model_251 INPUT,1.5V,FULLTERM, 9MA,IND,10%
Model_61 3-STATE,1.8V,SLOWEST, 8MA,IND,10%
Model_62 3-STATE,1.8V,SLOWEST, 5MA,IND,10%
Model_63 3-STATE,1.8V,slow, 7MA,IND,10%
Model_64 3-STATE,1.8V,slow, 6MA,IND,10%
Model_65 3-STATE,1.8V,SLOWEST, 9MA,IND,10%
Model_66 3-STATE,1.8V,slow, 11MA,IND,10%
Model_67 3-STATE,1.8V,SLOWEST, 12MA,IND,10%
Model_68 3-STATE,1.8V,SLOWEST, 7MA,IND,10%
Model_69 3-STATE,1.8V,slow, 10MA,IND,10%
Model_70 3-STATE,1.8V,SLOWEST, 6MA,IND,10%
Model_71 3-STATE,1.8V,slow, 8MA,IND,10%
Model_72 3-STATE,1.8V,slow, 5MA,IND,10%
Model_73 3-STATE,1.8V,SLOWEST, 11MA,IND,10%
Model_74 3-STATE,1.8V,SLOWEST, 10MA,IND,10%
Model_75 3-STATE,1.8V,slow, 9MA,IND,10%
Model_76 3-STATE,1.8V,slow, 12MA,IND,10%
Model_93 3-STATE,1.5V,SLOWEST, 8MA,IND,10%
Model_94 3-STATE,1.5V,SLOWEST, 5MA,IND,10%
Model_95 3-STATE,1.5V,slow, 7MA,IND,10%
Model_96 3-STATE,1.5V,slow, 6MA,IND,10%
Model_97 3-STATE,1.5V,SLOWEST, 9MA,IND,10%
Model_98 3-STATE,1.5V,slow, 11MA,IND,10%
Model_99 3-STATE,1.5V,SLOWEST, 12MA,IND,10%
|   Usage OUTPUT#1.8/3.3#X#X#BC1833DV40DCPBFBP18LL_SSDHH.PAD
|   Base model BC1833DV40DCPBFBP18LL_SSDHH
[Model Selector] Selector_3
Model_13 I/O,1.8V,Pull-up/down off,slow,IND,10%
Model_14 I/O,1.8V,Pull-down,fast,IND,10%
Model_15 I/O,1.8V,Pull-down,slow,IND,10%
Model_16 I/O,1.8V,Pull-up,fast,IND,10%
Model_17 I/O,1.8V,Pull-up/down off,fast,IND,10%
Model_18 I/O,1.8V,Pull-up,slow,IND,10%
Model_19 I/O,3.3V,Pull-up/down off,slow,IND,10%
Model_20 I/O,3.3V,Pull-down,fast,IND,10%
Model_21 I/O,3.3V,Pull-down,slow,IND,10%
Model_22 I/O,3.3V,Pull-up,fast,IND,10%
Model_23 I/O,3.3V,Pull-up/down off,fast,IND,10%
Model_24 I/O,3.3V,Pull-up,slow,IND,10%
|   Usage I/O#1.8/3.3#X#X#BC1833DV40DCPBFBP18LL_SSDHH.PAD
|   Base model BC1833DV40DCPBFBP18LL_SSDHH
[Model Selector] Selector_4
Model_13 I/O,1.8V,Pull-up/down off,slow,IND,10%
Model_14 I/O,1.8V,Pull-down,fast,IND,10%
Model_15 I/O,1.8V,Pull-down,slow,IND,10%
Model_16 I/O,1.8V,Pull-up,fast,IND,10%
Model_17 I/O,1.8V,Pull-up/down off,fast,IND,10%
Model_18 I/O,1.8V,Pull-up,slow,IND,10%
Model_19 I/O,3.3V,Pull-up/down off,slow,IND,10%
Model_20 I/O,3.3V,Pull-down,fast,IND,10%
Model_21 I/O,3.3V,Pull-down,slow,IND,10%
Model_22 I/O,3.3V,Pull-up,fast,IND,10%
Model_23 I/O,3.3V,Pull-up/down off,fast,IND,10%
Model_24 I/O,3.3V,Pull-up,slow,IND,10%
|   Usage I/O#1.5/1.8#X#X#BCSHTLTCSCDDVPBFZ_SSGFV.PAD
|   Base model BCSHTLTCSCDDVPBFZ_SSGFV
[Model Selector] Selector_5
Model_271 3-STATE,1.8V,SLOWEST, 8MA,IND,10%
Model_272 3-STATE,1.8V,SLOWEST, 5MA,IND,10%
Model_273 3-STATE,1.8V,slow, 7MA,IND,10%
Model_274 3-STATE,1.8V,slow, 6MA,IND,10%
Model_275 3-STATE,1.8V,SLOWEST, 9MA,IND,10%
Model_276 3-STATE,1.8V,slow, 11MA,IND,10%
Model_277 3-STATE,1.8V,SLOWEST, 12MA,IND,10%
Model_278 3-STATE,1.8V,SLOWEST, 7MA,IND,10%
Model_279 3-STATE,1.8V,slow, 10MA,IND,10%
Model_280 3-STATE,1.8V,SLOWEST, 6MA,IND,10%
Model_281 3-STATE,1.8V,slow, 8MA,IND,10%
Model_282 3-STATE,1.8V,slow, 5MA,IND,10%
Model_283 3-STATE,1.8V,SLOWEST, 11MA,IND,10%
Model_284 3-STATE,1.8V,SLOWEST, 10MA,IND,10%
Model_285 3-STATE,1.8V,slow, 9MA,IND,10%
Model_286 3-STATE,1.8V,slow, 12MA,IND,10%
Model_303 3-STATE,1.5V,SLOWEST, 8MA,IND,10%
Model_304 3-STATE,1.5V,SLOWEST, 5MA,IND,10%
Model_305 3-STATE,1.5V,slow, 7MA,IND,10%
Model_306 3-STATE,1.5V,slow, 6MA,IND,10%
Model_307 3-STATE,1.5V,SLOWEST, 9MA,IND,10%
Model_308 3-STATE,1.5V,slow, 11MA,IND,10%
Model_309 3-STATE,1.5V,SLOWEST, 12MA,IND,10%
Model_310 3-STATE,1.5V,SLOWEST, 7MA,IND,10%
Model_311 3-STATE,1.5V,slow, 10MA,IND,10%
Model_312 3-STATE,1.5V,SLOWEST, 6MA,IND,10%
Model_313 3-STATE,1.5V,slow, 8MA,IND,10%
Model_314 3-STATE,1.5V,slow, 5MA,IND,10%
Model_315 3-STATE,1.5V,SLOWEST, 11MA,IND,10%
Model_316 3-STATE,1.5V,SLOWEST, 10MA,IND,10%
Model_317 3-STATE,1.5V,slow, 9MA,IND,10%
Model_318 3-STATE,1.5V,slow, 12MA,IND,10%
Model_335 3-STATE,1.8V,fast, 12MA,IND,10%
Model_336 3-STATE,1.8V,FASTEST, 5MA,IND,10%
Model_337 3-STATE,1.8V,FASTEST, 9MA,IND,10%
Model_338 3-STATE,1.8V,fast, 5MA,IND,10%
Model_339 3-STATE,1.8V,FASTEST, 7MA,IND,10%
Model_340 3-STATE,1.8V,FASTEST, 6MA,IND,10%
Model_341 3-STATE,1.8V,fast, 9MA,IND,10%
Model_342 3-STATE,1.8V,FASTEST, 11MA,IND,10%
Model_343 3-STATE,1.8V,fast, 7MA,IND,10%
Model_344 3-STATE,1.8V,FASTEST, 10MA,IND,10%
Model_345 3-STATE,1.8V,fast, 6MA,IND,10%
Model_346 3-STATE,1.8V,FASTEST, 8MA,IND,10%
Model_347 3-STATE,1.8V,fast, 11MA,IND,10%
Model_348 3-STATE,1.8V,fast, 10MA,IND,10%
Model_349 3-STATE,1.8V,FASTEST, 12MA,IND,10%
Model_350 3-STATE,1.8V,fast, 8MA,IND,10%
Model_367 3-STATE,1.5V,fast, 12MA,IND,10%
Model_368 3-STATE,1.5V,FASTEST, 5MA,IND,10%
Model_369 3-STATE,1.5V,FASTEST, 9MA,IND,10%
Model_370 3-STATE,1.5V,fast, 5MA,IND,10%
Model_371 3-STATE,1.5V,FASTEST, 7MA,IND,10%
Model_372 3-STATE,1.5V,FASTEST, 6MA,IND,10%
Model_373 3-STATE,1.5V,fast, 9MA,IND,10%
Model_374 3-STATE,1.5V,FASTEST, 11MA,IND,10%
Model_375 3-STATE,1.5V,fast, 7MA,IND,10%
Model_376 3-STATE,1.5V,FASTEST, 10MA,IND,10%
Model_377 3-STATE,1.5V,fast, 6MA,IND,10%
Model_378 3-STATE,1.5V,FASTEST, 8MA,IND,10%
Model_379 3-STATE,1.5V,fast, 11MA,IND,10%
Model_380 3-STATE,1.5V,fast, 10MA,IND,10%
Model_381 3-STATE,1.5V,FASTEST, 12MA,IND,10%
Model_382 3-STATE,1.5V,fast, 8MA,IND,10%
Model_399 3-STATE,1.8V,SLOWEST, 8MA,IND,10%
Model_400 3-STATE,1.8V,SLOWEST, 5MA,IND,10%
Model_401 3-STATE,1.8V,slow, 7MA,IND,10%
Model_402 3-STATE,1.8V,slow, 6MA,IND,10%
Model_403 3-STATE,1.8V,SLOWEST, 9MA,IND,10%
Model_404 3-STATE,1.8V,slow, 11MA,IND,10%
Model_405 3-STATE,1.8V,SLOWEST, 12MA,IND,10%
Model_406 3-STATE,1.8V,SLOWEST, 7MA,IND,10%
Model_407 3-STATE,1.8V,slow, 10MA,IND,10%
Model_408 3-STATE,1.8V,SLOWEST, 6MA,IND,10%
Model_409 3-STATE,1.8V,slow, 8MA,IND,10%
Model_410 3-STATE,1.8V,slow, 5MA,IND,10%
Model_411 3-STATE,1.8V,SLOWEST, 11MA,IND,10%
Model_412 3-STATE,1.8V,SLOWEST, 10MA,IND,10%
Model_413 3-STATE,1.8V,slow, 9MA,IND,10%
Model_414 3-STATE,1.8V,slow, 12MA,IND,10%
Model_431 3-STATE,1.5V,SLOWEST, 8MA,IND,10%
Model_432 3-STATE,1.5V,SLOWEST, 5MA,IND,10%
Model_433 3-STATE,1.5V,slow, 7MA,IND,10%
Model_434 3-STATE,1.5V,slow, 6MA,IND,10%
Model_435 3-STATE,1.5V,SLOWEST, 9MA,IND,10%
Model_436 3-STATE,1.5V,slow, 11MA,IND,10%
Model_437 3-STATE,1.5V,SLOWEST, 12MA,IND,10%
Model_438 3-STATE,1.5V,SLOWEST, 7MA,IND,10%
Model_439 3-STATE,1.5V,slow, 10MA,IND,10%
Model_440 3-STATE,1.5V,SLOWEST, 6MA,IND,10%
Model_441 3-STATE,1.5V,slow, 8MA,IND,10%
Model_442 3-STATE,1.5V,slow, 5MA,IND,10%
Model_443 3-STATE,1.5V,SLOWEST, 11MA,IND,10%
Model_444 3-STATE,1.5V,SLOWEST, 10MA,IND,10%
Model_445 3-STATE,1.5V,slow, 9MA,IND,10%
Model_446 3-STATE,1.5V,slow, 12MA,IND,10%
Model_463 3-STATE,1.8V,fast, 12MA,IND,10%
Model_464 3-STATE,1.8V,FASTEST, 5MA,IND,10%
Model_465 3-STATE,1.8V,FASTEST, 9MA,IND,10%
Model_466 3-STATE,1.8V,fast, 5MA,IND,10%
Model_467 3-STATE,1.8V,FASTEST, 7MA,IND,10%
Model_468 3-STATE,1.8V,FASTEST, 6MA,IND,10%
Model_469 3-STATE,1.8V,fast, 9MA,IND,10%
Model_470 3-STATE,1.8V,FASTEST, 11MA,IND,10%
Model_471 3-STATE,1.8V,fast, 7MA,IND,10%
Model_472 3-STATE,1.8V,FASTEST, 10MA,IND,10%
Model_473 3-STATE,1.8V,fast, 6MA,IND,10%
Model_474 3-STATE,1.8V,FASTEST, 8MA,IND,10%
Model_475 3-STATE,1.8V,fast, 11MA,IND,10%
Model_476 3-STATE,1.8V,fast, 10MA,IND,10%
Model_477 3-STATE,1.8V,FASTEST, 12MA,IND,10%
Model_478 3-STATE,1.8V,fast, 8MA,IND,10%
Model_495 3-STATE,1.5V,fast, 12MA,IND,10%
Model_496 3-STATE,1.5V,FASTEST, 5MA,IND,10%
Model_497 3-STATE,1.5V,FASTEST, 9MA,IND,10%
Model_498 3-STATE,1.5V,fast, 5MA,IND,10%
Model_499 3-STATE,1.5V,FASTEST, 7MA,IND,10%
Model_500 3-STATE,1.5V,FASTEST, 6MA,IND,10%
Model_501 3-STATE,1.5V,fast, 9MA,IND,10%
Model_502 3-STATE,1.5V,FASTEST, 11MA,IND,10%
Model_503 3-STATE,1.5V,fast, 7MA,IND,10%
Model_504 3-STATE,1.5V,FASTEST, 10MA,IND,10%
Model_505 3-STATE,1.5V,fast, 6MA,IND,10%
Model_506 3-STATE,1.5V,FASTEST, 8MA,IND,10%
Model_507 3-STATE,1.5V,fast, 11MA,IND,10%
Model_508 3-STATE,1.5V,fast, 10MA,IND,10%
Model_509 3-STATE,1.5V,FASTEST, 12MA,IND,10%
Model_510 3-STATE,1.5V,fast, 8MA,IND,10%
Model_527 INPUT,1.8V,HALFTERM, 12MA,IND,10%
Model_528 INPUT,1.8V,Pull-up/down off,IND,10%
Model_529 INPUT,1.8V,Pull-down,IND,10%
Model_530 INPUT,1.8V,FULLTERM, 5MA,IND,10%
Model_531 INPUT,1.8V,HALFTERM, 5MA,IND,10%
Model_532 INPUT,1.8V,Pull-up,IND,10%
Model_533 INPUT,1.8V,FULLTERM, 9MA,IND,10%
Model_534 INPUT,1.8V,FULLTERM, 7MA,IND,10%
Model_535 INPUT,1.8V,HALFTERM, 9MA,IND,10%
Model_536 INPUT,1.8V,FULLTERM, 6MA,IND,10%
Model_537 INPUT,1.8V,HALFTERM, 7MA,IND,10%
Model_538 INPUT,1.8V,HALFTERM, 6MA,IND,10%
Model_539 INPUT,1.8V,FULLTERM, 11MA,IND,10%
Model_540 INPUT,1.8V,Pull-up/down off,IND,10%
Model_541 INPUT,1.8V,FULLTERM, 10MA,IND,10%
Model_542 INPUT,1.8V,HALFTERM, 11MA,IND,10%
Model_543 INPUT,1.8V,FULLTERM, 8MA,IND,10%
Model_544 INPUT,1.8V,HALFTERM, 10MA,IND,10%
Model_545 INPUT,1.8V,Pull-down,IND,10%
Model_546 INPUT,1.8V,HALFTERM, 8MA,IND,10%
Model_547 INPUT,1.8V,Pull-up,IND,10%
Model_548 INPUT,1.8V,FULLTERM, 12MA,IND,10%
Model_571 INPUT,1.5V,FULLTERM, 7MA,IND,10%
Model_572 INPUT,1.5V,FULLTERM, 6MA,IND,10%
Model_573 INPUT,1.5V,HALFTERM, 12MA,IND,10%
Model_574 INPUT,1.5V,FULLTERM, 5MA,IND,10%
Model_575 INPUT,1.5V,Pull-up,IND,10%
Model_576 INPUT,1.5V,HALFTERM, 11MA,IND,10%
Model_577 INPUT,1.5V,HALFTERM, 10MA,IND,10%
Model_578 INPUT,1.5V,HALFTERM, 8MA,IND,10%
Model_579 INPUT,1.5V,FULLTERM, 12MA,IND,10%
Model_580 INPUT,1.5V,HALFTERM, 9MA,IND,10%
Model_581 INPUT,1.5V,Pull-up/down off,IND,10%
Model_582 INPUT,1.5V,HALFTERM, 7MA,IND,10%
Model_583 INPUT,1.5V,HALFTERM, 6MA,IND,10%
Model_584 INPUT,1.5V,FULLTERM, 11MA,IND,10%
Model_585 INPUT,1.5V,FULLTERM, 10MA,IND,10%
Model_586 INPUT,1.5V,Pull-down,IND,10%
Model_587 INPUT,1.5V,FULLTERM, 8MA,IND,10%
Model_588 INPUT,1.5V,HALFTERM, 5MA,IND,10%
Model_589 INPUT,1.5V,FULLTERM, 9MA,IND,10%
|   Usage INPUT#1.8/3.3#X#X#BC1833DV40DCPBFBP18LL_SSDHV.PAD
|   Base model BC1833DV40DCPBFBP18LL_SSDHV
[Model Selector] Selector_6
Model_625 I/O,1.8V,Pull-up/down off,slow,IND,10%
Model_626 I/O,1.8V,Pull-down,fast,IND,10%
Model_627 I/O,1.8V,Pull-down,slow,IND,10%
Model_628 I/O,1.8V,Pull-up,fast,IND,10%
Model_629 I/O,1.8V,Pull-up/down off,fast,IND,10%
Model_630 I/O,1.8V,Pull-up,slow,IND,10%
Model_631 I/O,3.3V,Pull-up/down off,slow,IND,10%
Model_632 I/O,3.3V,Pull-down,fast,IND,10%
Model_633 I/O,3.3V,Pull-down,slow,IND,10%
Model_634 I/O,3.3V,Pull-up,fast,IND,10%
Model_635 I/O,3.3V,Pull-up/down off,fast,IND,10%
Model_636 I/O,3.3V,Pull-up,slow,IND,10%
|   Usage I/O#1.8/3.3#X#X#BC1833DV40DCMLBPBFBP18LL_SSDHH.PAD
|   Base model BC1833DV40DCMLBPBFBP18LL_SSDHH
[Model Selector] Selector_7
Model_49 I/O,1.8V,Pull-up/down off,slow,IND,10%
Model_50 I/O,1.8V,Pull-down,fast,IND,10%
Model_51 I/O,1.8V,Pull-down,slow,IND,10%
Model_52 I/O,1.8V,Pull-up,fast,IND,10%
Model_53 I/O,1.8V,Pull-up/down off,fast,IND,10%
Model_54 I/O,1.8V,Pull-up,slow,IND,10%
Model_55 I/O,3.3V,Pull-up/down off,slow,IND,10%
Model_56 I/O,3.3V,Pull-down,fast,IND,10%
Model_57 I/O,3.3V,Pull-down,slow,IND,10%
Model_58 I/O,3.3V,Pull-up,fast,IND,10%
Model_59 I/O,3.3V,Pull-up/down off,fast,IND,10%
Model_60 I/O,3.3V,Pull-up,slow,IND,10%
|   Usage INPUT#1.8/3.3#X#X#IQ1833DVTCKPBFBP18LL_SSDHH.PAD
|   Base model IQ1833DVTCKPBFBP18LL_SSDHH
[Model Selector] Selector_8
Model_31 INPUT,1.8V,Pull-down,IND,10%
Model_32 INPUT,1.8V,Pull-up,IND,10%
Model_33 INPUT,1.8V,Pull-up/down off,IND,10%
Model_34 INPUT,3.3V,Pull-down,IND,10%
Model_35 INPUT,3.3V,Pull-up,IND,10%
Model_36 INPUT,3.3V,Pull-up/down off,IND,10%
|   Usage OUTPUT#1.5/1.8#X#X#BCSHTLTCSCDVPBFZ_SSGFV.PAD
|   Base model BCSHTLTCSCDVPBFZ_SSGFV
[Model Selector] Selector_9
Model_100 3-STATE,1.5V,SLOWEST, 7MA,IND,10%
Model_101 3-STATE,1.5V,slow, 10MA,IND,10%
Model_102 3-STATE,1.5V,SLOWEST, 6MA,IND,10%
Model_103 3-STATE,1.5V,slow, 8MA,IND,10%
Model_104 3-STATE,1.5V,slow, 5MA,IND,10%
Model_105 3-STATE,1.5V,SLOWEST, 11MA,IND,10%
Model_106 3-STATE,1.5V,SLOWEST, 10MA,IND,10%
Model_107 3-STATE,1.5V,slow, 9MA,IND,10%
Model_108 3-STATE,1.5V,slow, 12MA,IND,10%
Model_125 3-STATE,1.8V,fast, 12MA,IND,10%
Model_126 3-STATE,1.8V,FASTEST, 5MA,IND,10%
Model_127 3-STATE,1.8V,FASTEST, 9MA,IND,10%
Model_128 3-STATE,1.8V,fast, 5MA,IND,10%
Model_129 3-STATE,1.8V,FASTEST, 7MA,IND,10%
Model_130 3-STATE,1.8V,FASTEST, 6MA,IND,10%
Model_131 3-STATE,1.8V,fast, 9MA,IND,10%
Model_132 3-STATE,1.8V,FASTEST, 11MA,IND,10%
Model_133 3-STATE,1.8V,fast, 7MA,IND,10%
Model_134 3-STATE,1.8V,FASTEST, 10MA,IND,10%
Model_135 3-STATE,1.8V,fast, 6MA,IND,10%
Model_136 3-STATE,1.8V,FASTEST, 8MA,IND,10%
Model_137 3-STATE,1.8V,fast, 11MA,IND,10%
Model_138 3-STATE,1.8V,fast, 10MA,IND,10%
Model_139 3-STATE,1.8V,FASTEST, 12MA,IND,10%
Model_140 3-STATE,1.8V,fast, 8MA,IND,10%
Model_157 3-STATE,1.5V,fast, 12MA,IND,10%
Model_158 3-STATE,1.5V,FASTEST, 5MA,IND,10%
Model_159 3-STATE,1.5V,FASTEST, 9MA,IND,10%
Model_160 3-STATE,1.5V,fast, 5MA,IND,10%
Model_161 3-STATE,1.5V,FASTEST, 7MA,IND,10%
Model_162 3-STATE,1.5V,FASTEST, 6MA,IND,10%
Model_163 3-STATE,1.5V,fast, 9MA,IND,10%
Model_164 3-STATE,1.5V,FASTEST, 11MA,IND,10%
Model_165 3-STATE,1.5V,fast, 7MA,IND,10%
Model_166 3-STATE,1.5V,FASTEST, 10MA,IND,10%
Model_167 3-STATE,1.5V,fast, 6MA,IND,10%
Model_168 3-STATE,1.5V,FASTEST, 8MA,IND,10%
Model_169 3-STATE,1.5V,fast, 11MA,IND,10%
Model_170 3-STATE,1.5V,fast, 10MA,IND,10%
Model_171 3-STATE,1.5V,FASTEST, 12MA,IND,10%
Model_172 3-STATE,1.5V,fast, 9MA,IND,10%
Model_61 3-STATE,1.8V,SLOWEST, 8MA,IND,10%
Model_62 3-STATE,1.8V,SLOWEST, 5MA,IND,10%
Model_63 3-STATE,1.8V,slow, 7MA,IND,10%
Model_64 3-STATE,1.8V,slow, 6MA,IND,10%
Model_65 3-STATE,1.8V,SLOWEST, 9MA,IND,10%
Model_66 3-STATE,1.8V,slow, 11MA,IND,10%
Model_67 3-STATE,1.8V,SLOWEST, 12MA,IND,10%
Model_68 3-STATE,1.8V,SLOWEST, 7MA,IND,10%
Model_69 3-STATE,1.8V,slow, 10MA,IND,10%
Model_70 3-STATE,1.8V,SLOWEST, 6MA,IND,10%
Model_71 3-STATE,1.8V,slow, 8MA,IND,10%
Model_72 3-STATE,1.8V,slow, 5MA,IND,10%
Model_73 3-STATE,1.8V,SLOWEST, 11MA,IND,10%
Model_74 3-STATE,1.8V,SLOWEST, 10MA,IND,10%
Model_75 3-STATE,1.8V,slow, 9MA,IND,10%
Model_76 3-STATE,1.8V,slow, 12MA,IND,10%
Model_93 3-STATE,1.5V,SLOWEST, 8MA,IND,10%
Model_94 3-STATE,1.5V,SLOWEST, 5MA,IND,10%
Model_95 3-STATE,1.5V,slow, 7MA,IND,10%
Model_96 3-STATE,1.5V,slow, 6MA,IND,10%
Model_97 3-STATE,1.5V,SLOWEST, 9MA,IND,10%
Model_98 3-STATE,1.5V,slow, 11MA,IND,10%
Model_99 3-STATE,1.5V,SLOWEST, 12MA,IND,10%
|   Usage OUTPUT#1.8/3.3#X#X#BC1833DV40DCPBFBP18LL_SSDHV.PAD
|   Base model BC1833DV40DCPBFBP18LL_SSDHV
[Model Selector] Selector_10
Model_625 I/O,1.8V,Pull-up/down off,slow,IND,10%
Model_626 I/O,1.8V,Pull-down,fast,IND,10%
Model_627 I/O,1.8V,Pull-down,slow,IND,10%
Model_628 I/O,1.8V,Pull-up,fast,IND,10%
Model_629 I/O,1.8V,Pull-up/down off,fast,IND,10%
Model_630 I/O,1.8V,Pull-up,slow,IND,10%
Model_631 I/O,3.3V,Pull-up/down off,slow,IND,10%
Model_632 I/O,3.3V,Pull-down,fast,IND,10%
Model_633 I/O,3.3V,Pull-down,slow,IND,10%
Model_634 I/O,3.3V,Pull-up,fast,IND,10%
Model_635 I/O,3.3V,Pull-up/down off,fast,IND,10%
Model_636 I/O,3.3V,Pull-up,slow,IND,10%
|   Usage I/O#1.8/3.3#X#X#BC1833DV40DCPBFBP18LL_SSDHV.PAD
|   Base model BC1833DV40DCPBFBP18LL_SSDHV
[Model Selector] Selector_11
Model_625 I/O,1.8V,Pull-up/down off,slow,IND,10%
Model_626 I/O,1.8V,Pull-down,fast,IND,10%
Model_627 I/O,1.8V,Pull-down,slow,IND,10%
Model_628 I/O,1.8V,Pull-up,fast,IND,10%
Model_629 I/O,1.8V,Pull-up/down off,fast,IND,10%
Model_630 I/O,1.8V,Pull-up,slow,IND,10%
Model_631 I/O,3.3V,Pull-up/down off,slow,IND,10%
Model_632 I/O,3.3V,Pull-down,fast,IND,10%
Model_633 I/O,3.3V,Pull-down,slow,IND,10%
Model_634 I/O,3.3V,Pull-up,fast,IND,10%
Model_635 I/O,3.3V,Pull-up/down off,fast,IND,10%
Model_636 I/O,3.3V,Pull-up,slow,IND,10%
|   Usage INPUT#1.8/3.3#X#X#IHHV1833DVHYP18LL_SSDHH.PAD
|   Base model IHHV1833DVHYP18LL_SSDHH
[Model Selector] Selector_12
Model_611 INPUT,1.8V,NORMAL,IND,10%
Model_612 INPUT,3.3V,NORMAL,IND,10%
| Models and submodels in the file (318): Model_13 (I/O), Model_14 (I/O), Model_15 (I/O), Model_16 (I/O), Model_17 (I/O), Model_18 (I/O), Model_19 (I/O), Model_20 (I/O), Model_21 (I/O), Model_22 (I/O), Model_23 (I/O), Model_24 (I/O), Model_31 (Input), Model_32 (Input), Model_33 (Input), Model_34 (Input), Model_35 (Input), Model_36 (Input), Model_49 (I/O), Model_50 (I/O), Model_51 (I/O), Model_52 (I/O), Model_53 (I/O), Model_54 (I/O), Model_55 (I/O), Model_56 (I/O), Model_57 (I/O), Model_58 (I/O), Model_59 (I/O), Model_60 (I/O), Model_61 (3-state), Model_62 (3-state), Model_63 (3-state), Model_64 (3-state), Model_65 (3-state), Model_66 (3-state), Model_67 (3-state), Model_68 (3-state), Model_69 (3-state), Model_70 (3-state), Model_71 (3-state), Model_72 (3-state), Model_73 (3-state), Model_74 (3-state), Model_75 (3-state), Model_76 (3-state), Model_93 (3-state), Model_94 (3-state), Model_95 (3-state), Model_96 (3-state), Model_97 (3-state), Model_98 (3-state), Model_99 (3-state), Model_100 (3-state), Model_101 (3-state), Model_102 (3-state), Model_103 (3-state), Model_104 (3-state), Model_105 (3-state), Model_106 (3-state), Model_107 (3-state), Model_108 (3-state), Model_125 (3-state), Model_126 (3-state), Model_127 (3-state), Model_128 (3-state), Model_129 (3-state), Model_130 (3-state), Model_131 (3-state), Model_132 (3-state), Model_133 (3-state), Model_134 (3-state), Model_135 (3-state), Model_136 (3-state), Model_137 (3-state), Model_138 (3-state), Model_139 (3-state), Model_140 (3-state), Model_157 (3-state), Model_158 (3-state)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
